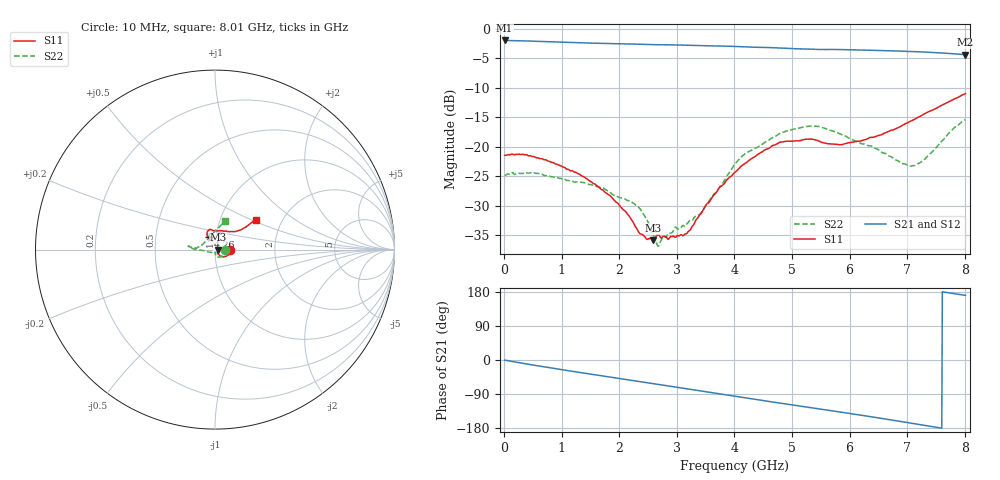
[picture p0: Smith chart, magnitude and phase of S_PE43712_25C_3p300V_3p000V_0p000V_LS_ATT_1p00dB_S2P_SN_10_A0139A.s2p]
! DEVICE ID: PE43712
! File Path: z:\PE43713\PE43713_CHAR_NOM_04292014\AMB\3p300\LS_ATT_1p00dB\PE43713_AMB_3p300V_3p000V_0p000V_LS_ATT_1p00dB_S2P_SN_10_A0139A.s2p
! Serial: 10
! Lot: A0139A
! Temp: 25C
! VDD: 3.300
! VSS: 0.000
! Control_Hi: 3.000
! Control_Lo: 0.000
! Attenuation Step: 1.00dB
! Port 1: RF1
! Port 2: RF2
! ThroughPath:1-2
! IDD: 0.0001469298
! ISS: -1.47e-007
#  Hz  S  RI  R  50
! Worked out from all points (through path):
!   801 points, 10 MHz to 8.01 GHz, reference 50 ohm
!   highest |S21| = -2.01 dB at 10 MHz (marker M1); lowest = -4.4 dB at 8.01 GHz (marker M2)
!   group delay of S21, straight-line fit = 64.8 ps
!   lowest |S11| = -35.8 dB at 2.59 GHz (marker M3), VSWR 1.03, Z = 51.6 - j4.67e-05 ohm
!   |S11| at or under -10 dB: start of sweep to end of sweep
!   |S22| runs from -36.8 to -15.4 dB; largest |S21 - S12| = 0.0024
!   S11 on the Smith chart (normalised r, x): 10 MHz: 1.19, -0.00; 4.26 GHz: 0.92, +0.13; 8.01 GHz: 1.47, +0.53
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1e7  0.0847 -0.000485  0.7937 -0.00427  0.7938 -0.00412  0.0574 -0.000611
6.8e8  0.0714 -0.0319  0.7405 -0.236  0.7402 -0.2358  0.0499 -0.0288
1.35e9  0.0401 -0.04  0.6304 -0.4205  0.63 -0.4203  0.0265 -0.0422
1.86e9  0.0235 -0.0296  0.523 -0.5328  0.5228 -0.5325  0.0122 -0.0385
2.14e9  0.0157 -0.022  0.4559 -0.5848  0.4558 -0.5845  0.00329 -0.0349
2.29e9  0.015 -0.0144  0.4175 -0.6091  0.4177 -0.6089  0.00351 -0.0319
2.47e9  0.0152 -0.00682  0.3701 -0.6347  0.3702 -0.6346  0.00177 -0.0244
2.59e9  0.0162 -4.52e-07  0.338 -0.6486  0.338 -0.6488  0.00174 -0.018
2.68e9  0.0173 0.00469  0.3148 -0.659  0.315 -0.6587  0.00497 -0.0135
2.86e9  0.0137 0.00939  0.2649 -0.679  0.2649 -0.6792  -0.000637 -0.0184
3.19e9  0.00432 0.0185  0.1692 -0.7031  0.1693 -0.703  -0.0154 -0.0166
3.43e9  0.000673 0.0276  0.0986 -0.7106  0.099 -0.7109  -0.0233 -0.0153
3.74e9  -0.00884 0.0443  0.00903 -0.7128  0.00968 -0.7126  -0.0438 -0.0108
4.01e9  -0.0226 0.0565  -0.0701 -0.703  -0.0696 -0.7027  -0.0713 -0.00462
4.26e9  -0.0359 0.0682  -0.1391 -0.6846  -0.1389 -0.6845  -0.0915 -0.000529
4.79e9  -0.043 0.1005  -0.2762 -0.6265  -0.2757 -0.6267  -0.1292 0.00699
5.35e9  -0.0276 0.1123  -0.3961 -0.5395  -0.396 -0.5389  -0.1494 0.0181
5.85e9  0.00834 0.1037  -0.4905 -0.4485  -0.4896 -0.4486  -0.1267 0.0127
6.68e9  0.0905 0.1002  -0.5981 -0.2514  -0.5979 -0.251  -0.0814 0.0191
7.03e9  0.124 0.1039  -0.6223 -0.1577  -0.6218 -0.1578  -0.0536 0.0437
7.16e9  0.1371 0.1081  -0.6269 -0.1218  -0.626 -0.1217  -0.0406 0.0583
8.01e9  0.227 0.1664  -0.5939 0.0983  -0.5922 0.0973  0.0551 0.1608
